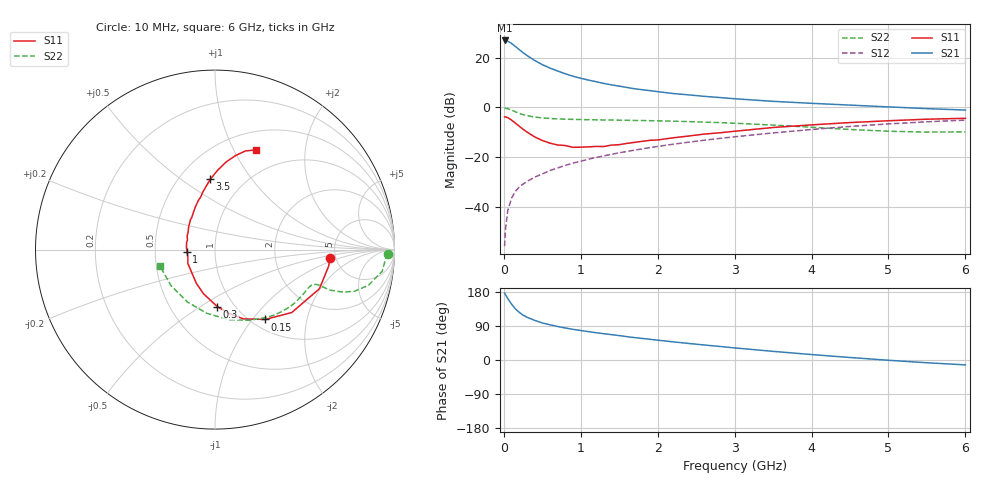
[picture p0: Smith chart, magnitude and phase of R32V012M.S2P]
! SIEMENS Small Signal Semiconductors
! BFR181
! Si NPN RF Bipolar Junction Transistor in SOT23
! VCE = 2 V  IC = 12 mA
! Common Emitter S-Parameters:  May  1996
# GHz  S  MA  R  50
!  f  S11  S21  S12  S22
! GHz  MAG  ANG  MAG  ANG  MAG  ANG  MAG  ANG
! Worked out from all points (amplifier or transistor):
!   36 points, 10 MHz to 6 GHz, reference 50 ohm
!   highest |S21| = 26.9 dB at 10 MHz (marker M1)
!   |S21| within 3 dB of that: start of sweep to 172.9 MHz
!   unconditionally stable (mu >= 1): 498.9 MHz to 2.763 GHz
!   at 250 MHz: K = 0.73, MSG = 26.5 dB, |S12| = -30.9 dB
!   at 1.4 GHz: K = 1.12, MAG = 11.9 dB, |S12| = -18.9 dB
!   at 6 GHz: K = 0.88, MSG = 2.0 dB, |S12| = -5.2 dB
!   S11 on the Smith chart (normalised r, x): 10 MHz: 4.45, -0.75; 150 MHz: 1.15, -1.16; 300 MHz: 0.84, -0.59; 1 GHz: 0.73, -0.02; 3.5 GHz: 0.70, +0.65; 6 GHz: 0.71, +1.23
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0.01  0.6417 -4.4  22.17 176.3  0.0016 85.0  0.963 -1.4
0.02  0.6398 -8.3  21.92 172.7  0.0033 88.4  0.9524 -3.0
0.05  0.6214 -20.5  21.43 162.6  0.0082 80.1  0.9394 -7.4
0.1  0.5531 -39.3  19.3 147.6  0.0148 74.0  0.8778 -13.1
0.15  0.4794 -54.3  16.76 134.8  0.0203 69.6  0.8117 -16.6
0.2  0.4168 -67.8  14.53 125.7  0.0248 68.4  0.7548 -18.3
0.25  0.3617 -78.1  12.61 118.5  0.0285 66.6  0.7098 -19.0
0.3  0.3176 -87.7  11.06 112.9  0.0321 67.3  0.68 -19.4
0.4  0.254 -104.7  8.788 104.7  0.0392 67.7  0.6379 -19.1
0.5  0.2146 -118.9  7.21 97.8  0.0455 69.0  0.6108 -18.9
0.6  0.1895 -130.4  6.167 92.9  0.0533 69.8  0.5955 -19.0
0.7  0.1743 -143.2  5.369 88.4  0.0601 70.5  0.5846 -19.4
0.8  0.1698 -152.8  4.723 84.5  0.0676 70.6  0.5764 -19.9
1  0.1573 -176.1  3.839 77.8  0.0821 71.4  0.5667 -21.3
1.1  0.1598 174.6  3.531 74.9  0.0903 71.6  0.5624 -22.2
1.3  0.1623 160.9  3.021 69.4  0.1054 71.0  0.5558 -24.4
1.6  0.1877 142.0  2.507 61.6  0.1292 70.2  0.5473 -28.1
2.2  0.243 119.3  1.895 47.9  0.1804 67.1  0.5259 -37.0
3.5  0.3921 93.9  1.318 22.8  0.3049 56.0  0.4387 -64.0
4.5  0.4927 82.7  1.107 6.6  0.4113 44.0  0.3575 -97.5
5.5  0.5758 72.8  0.94 -7.3  0.51 29.9  0.3167 -140.6
6  0.6004 67.6  0.88 -12.9  0.5524 22.3  0.3204 -163.3
